PROGRAM IL
VAR
	RANGE_PG_PS1:RANGEJD;
	RANGE_PG_PS2:RANGEJD;
	RANGE_PG_PS3:RANGEJD;
	RANGE_PG_PS4:RANGEJD;
	RANGE_PG_PS5:RANGEJD;
	RANGE_PG_PS6:RANGEJD;
	RANGE_PG_PS7:RANGEJD;
	RANGE_PG_PS8:RANGEJD;
	RANGE_PG_PS9:RANGEJD;
	
	RANGE_MFC1:RANGEJD;
	RANGE_MFC2:RANGEJD;
	RANGE_MFC3:RANGEJD;
	RANGE_MFC4:RANGEJD;
	RANGE_MFC5:RANGEJD;
	RANGE_MFC6:RANGEJD;
	RANGE_MFC7:RANGEJD;
	RANGE_MFC8:RANGEJD;
	RANGE_MFC9:RANGEJD;
	
	RANGE_CHAMBER_HEATER1:RANGEJD;
	RANGE_CHAMBER_HEATER2:RANGEJD;
	RANGE_CHAMBER_HEATER3:RANGEJD;
	
	RANGE_LID_HEATER:RANGEJD;
	
	RANGE_STAGE1:RANGEJD;
	RANGE_STAGE2:RANGEJD;
	RANGE_STAGE3:RANGEJD;
	RANGE_STAGE4:RANGEJD;
	
	//INTERLOCK	
	TON_PrepareTransfer:TON;	
	TON_TransferWafer:TON;	
	TON_OpenGasValve:TON;	
	TON_CloseGasValve:TON;	
	TON_OpenCloseSlitValve:TON;
	
	ALWAYS_TRUE:BOOL:=TRUE;
END_VAR
VAR // added by the converter: edge detectors and wires of the graphical bodies
    _w1, _w2, _w3, _w4, _w5 : BOOL;
END_VAR

VALVE();
Temp();
SYS();
SPLC();
ACT_HEATER();
ACT_MFC();
ACT_PG_PS();

//TMP Pressure OUT OF RANGE
	IF GV.PMConfig.TurboN2Pressure	<=	GV.TurboN2PurgePressure
		THEN
		PM.INFO.Alarm.TurboN2PurgePressureOutOfRange:=TRUE;
		ELSE
		PM.INFO.Alarm.TurboN2PurgePressureOutOfRange:=FALSE;	
	END_IF
	
//PrepareTransfer TIMEOUT
	TON_PrepareTransfer(IN:= GV_IL.STATUS_PrepareTransfer, PT:=INT_TO_TIME(GV.PMConfig.PrepareTransferTimeout)*1000 , Q=> , ET=> );	
	IF TON_PrepareTransfer.Q
		THEN
		PM.INFO.Alarm.PrepareTransferTimerout:=TRUE;
		ELSE
		PM.INFO.Alarm.PrepareTransferTimerout:=FALSE;
	END_IF
	
//TransferWafer TIMEOUT
	TON_TransferWafer(IN:=GV_IL.STATUS_TransferWafer , PT:= INT_TO_TIME(GV.PMConfig.TransferWaferTimeout)*1000, Q=> , ET=> );
	IF TON_TransferWafer.Q
		THEN
		PM.INFO.Alarm.TransferWaferTimeout:=TRUE;
		ELSE
		PM.INFO.Alarm.TransferWaferTimeout:=FALSE;	
	END_IF
	
//OpenGasValve TIMEOUT
	TON_OpenGasValve(IN:=GV_IL.STATUS_OpenGasValve , PT:= INT_TO_TIME(GV.PMConfig.OpenGasValveTimeout)*1000, Q=> , ET=> );
	IF TON_OpenGasValve.Q
		THEN
		PM.INFO.Alarm.OpenGasValveTimeout:=TRUE;
		ELSE 
		PM.INFO.Alarm.OpenGasValveTimeout:=FALSE;
	END_IF
	
//CloseGasValve TIMEOUT
	TON_CloseGasValve(IN:=GV_IL.STATUS_CloseGasValve , PT:= INT_TO_TIME(GV.PMConfig.CloseGasValveTimeout)*1000, Q=> , ET=> );
	IF TON_CloseGasValve.Q
		THEN
		PM.INFO.Alarm.CloseGasValveTimeout:=TRUE;
		ELSE
		PM.INFO.Alarm.CloseGasValveTimeout:=FALSE;
	END_IF
	
//OpenCloseSlitValve TIMEOUT
	TON_OpenCloseSlitValve(IN:=GV_IL.STATUS_OpenCloseSlitValve , PT:= INT_TO_TIME(GV.PMConfig.OpenCloseSlitValveTimeout)*1000, Q=> , ET=> );
	IF TON_OpenCloseSlitValve.Q
		THEN
		PM.INFO.Alarm.OpenCloseSlitValveTimeout:=TRUE;
		ELSE
		PM.INFO.Alarm.OpenCloseSlitValveTimeout:=FALSE;	
	END_IF
	
	
//PRESSURE ALARM
	//PM.INFO.Alarm.PRESSURE:=
	
//ALARM OR WARNING OCCUR
	GV.ALARM_OCC:=NOT (
				 	//PM.INFO.Alarm.PRESSURE
					PM.INFO.Alarm.MFC1	
				AND PM.INFO.Alarm.MFC2	
				AND	PM.INFO.Alarm.MFC3
				AND PM.INFO.Alarm.MFC4	
				AND PM.INFO.Alarm.MFC5	
				AND PM.INFO.Alarm.MFC6
				AND PM.INFO.Alarm.MFC7	
				AND PM.INFO.Alarm.MFC8	
				AND PM.INFO.Alarm.MFC9
				AND PM.INFO.Alarm.WALL_TEMP	
				AND PM.INFO.Alarm.LID_TEMP	
				AND PM.INFO.Alarm.STAGE_TEMP1
				AND PM.INFO.Alarm.STAGE_TEMP2
				AND PM.INFO.Alarm.STAGE_TEMP3
				AND PM.INFO.Alarm.STAGE_TEMP4
				//AND PM.INFO.Alarm.Gas1FlowPressureOutOfRange
				//AND PM.INFO.Alarm.Gas2FlowPressureOutOfRange
				//AND PM.INFO.Alarm.Gas3FlowPressureOutOfRange
				//AND PM.INFO.Alarm.Gas4FlowPressureOutOfRange
				//AND PM.INFO.Alarm.Gas5FlowPressureOutOfRange
				//AND PM.INFO.Alarm.Gas6FlowPressureOutOfRange
				//AND PM.INFO.Alarm.TurboN2PurgePressureOutOfRange
				//AND PM.INFO.Alarm.PrepareTransferTimerout
				//AND PM.INFO.Alarm.TransferWaferTimeout
				//AND PM.INFO.Alarm.OpenGasValveTimeout
				//AND PM.INFO.Alarm.CloseGasValveTimeout
				//AND PM.INFO.Alarm.OpenCloseSlitValveTimeout
				//AND PM.INFO.Alarm.ATMCheckTimeout
				//AND PM.INFO.Alarm.DRY_PUMP
				//AND PM.INFO.Alarm.PENDULUM_VALVE
				//AND PM.INFO.Alarm.TURBO_PUMP
				AND (PM.INFO.Alarm.TOLERANCE_PRESSURE				
				AND PM.INFO.Alarm.TOLERANCE_MFC1
				AND PM.INFO.Alarm.TOLERANCE_MFC2
				AND PM.INFO.Alarm.TOLERANCE_MFC3
				AND PM.INFO.Alarm.TOLERANCE_MFC4
				AND PM.INFO.Alarm.TOLERANCE_MFC5
				AND PM.INFO.Alarm.TOLERANCE_MFC6
				AND PM.INFO.Alarm.TOLERANCE_MFC7
				AND PM.INFO.Alarm.TOLERANCE_MFC8
				AND PM.INFO.Alarm.TOLERANCE_MFC9
				AND PM.INFO.Alarm.TOLERANCE_WALL_TEMP
				AND PM.INFO.Alarm.TOLERANCE_LID_TEMP
				AND PM.INFO.Alarm.TOLERANCE_STAGE_TEMP1
				AND PM.INFO.Alarm.TOLERANCE_STAGE_TEMP2
				AND PM.INFO.Alarm.TOLERANCE_STAGE_TEMP3
				AND PM.INFO.Alarm.TOLERANCE_STAGE_TEMP4)
				);

	GV.WARNING_OCC:=NOT (
					//PM.INFO.Warning.PRESSURE					
					PM.INFO.Warning.MFC1
				AND PM.INFO.Warning.MFC2
				AND PM.INFO.Warning.MFC3
				AND PM.INFO.Warning.MFC4
				AND PM.INFO.Warning.MFC5
				AND PM.INFO.Warning.MFC6
				AND PM.INFO.Warning.MFC7
				AND PM.INFO.Warning.MFC8
				AND PM.INFO.Warning.MFC9
				AND PM.INFO.Warning.WALL_TEMP
				AND PM.INFO.Warning.LID_TEMP
				AND PM.INFO.Warning.STAGE_TEMP1
				AND PM.INFO.Warning.STAGE_TEMP2
				AND PM.INFO.Warning.STAGE_TEMP3
				AND PM.INFO.Warning.STAGE_TEMP4
				//AND PM.INFO.Warning.Gas1FlowPressureOutOfRange
				//AND PM.INFO.Warning.Gas2FlowPressureOutOfRange
				//AND PM.INFO.Warning.Gas3FlowPressureOutOfRange
				//AND PM.INFO.Warning.Gas4FlowPressureOutOfRange
				//AND PM.INFO.Warning.Gas5FlowPressureOutOfRange
				//AND PM.INFO.Warning.Gas6FlowPressureOutOfRange
				//AND PM.INFO.Warning.OpenCloseSlitValveTimeout
				AND (PM.INFO.Warning.TOLERANCE_PRESSURE
				AND PM.INFO.Warning.TOLERANCE_MFC1
				AND PM.INFO.Warning.TOLERANCE_MFC2
				AND PM.INFO.Warning.TOLERANCE_MFC3
				AND PM.INFO.Warning.TOLERANCE_MFC4
				AND PM.INFO.Warning.TOLERANCE_MFC5
				AND PM.INFO.Warning.TOLERANCE_MFC6
				AND PM.INFO.Warning.TOLERANCE_MFC7
				AND PM.INFO.Warning.TOLERANCE_MFC8
				AND PM.INFO.Warning.TOLERANCE_MFC9
				AND PM.INFO.Warning.TOLERANCE_WALL_TEMP
				AND PM.INFO.Warning.TOLERANCE_LID_TEMP
				AND PM.INFO.Warning.TOLERANCE_STAGE_TEMP1
				AND PM.INFO.Warning.TOLERANCE_STAGE_TEMP2
				AND PM.INFO.Warning.TOLERANCE_STAGE_TEMP3
				AND PM.INFO.Warning.TOLERANCE_STAGE_TEMP4)
				);

ACTION ACT_HEATER:
//CHAMBER HEATER
	RANGE_CHAMBER_HEATER1(
	ENABLE:= GV.ChamberHeater.HeaterTolerance_Enable,
	SV:= REAL_TO_LREAL(GV.AO.Chamber_Temp1_SV),
	PV:= REAL_TO_LREAL( GV.AI.Chamber_Temp1), 
	RANGE_ALARM_H:= ANY_TO_REAL(GV.ChamberHeater.HeaterAlarmRange.SV), 
	RANGE_ALARM_L:= ANY_TO_LREAL(GV.ChamberHeater.HeaterAlarmRange.SV), 
	RANGE_WARNING_H:= ANY_TO_LREAL(GV.ChamberHeater.HeaterWarningRange.SV), 
	RANGE_WARNING_L:= ANY_TO_LREAL(GV.ChamberHeater.HeaterWarningRange.SV), 
	TIME_ALARM:= ANY_TO_LREAL(GV.ChamberHeater.HeaterAlarmTime.SV), 
	TIME_WARNING:= ANY_TO_LREAL(GV.ChamberHeater.HeaterWarningTime.SV), 
	ALARM=> , 
	WARNING=> );
	
	RANGE_CHAMBER_HEATER2(
	ENABLE:= GV.ChamberHeater.HeaterTolerance_Enable,
	SV:= REAL_TO_LREAL(GV.AO.Chamber_Temp2_SV),
	PV:= REAL_TO_LREAL( GV.AI.Chamber_Temp2), 
	RANGE_ALARM_H:= ANY_TO_LREAL(GV.ChamberHeater.HeaterAlarmRange.SV), 
	RANGE_ALARM_L:= ANY_TO_LREAL(GV.ChamberHeater.HeaterAlarmRange.SV), 
	RANGE_WARNING_H:= ANY_TO_LREAL(GV.ChamberHeater.HeaterWarningRange.SV), 
	RANGE_WARNING_L:= ANY_TO_LREAL(GV.ChamberHeater.HeaterWarningRange.SV), 
	TIME_ALARM:= ANY_TO_LREAL(GV.ChamberHeater.HeaterAlarmTime.SV), 
	TIME_WARNING:= ANY_TO_LREAL(GV.ChamberHeater.HeaterWarningTime.SV), 
	ALARM=> , 
	WARNING=> );
	
	RANGE_CHAMBER_HEATER3(
	ENABLE:= GV.ChamberHeater.HeaterTolerance_Enable,
	SV:= REAL_TO_LREAL(GV.AO.Chamber_Temp3_SV),
	PV:= REAL_TO_LREAL( GV.AI.Chamber_Temp3), 
	RANGE_ALARM_H:= ANY_TO_LREAL(GV.ChamberHeater.HeaterAlarmRange.SV), 
	RANGE_ALARM_L:= ANY_TO_LREAL(GV.ChamberHeater.HeaterAlarmRange.SV), 
	RANGE_WARNING_H:= ANY_TO_LREAL(GV.ChamberHeater.HeaterWarningRange.SV), 
	RANGE_WARNING_L:= ANY_TO_LREAL(GV.ChamberHeater.HeaterWarningRange.SV), 
	TIME_ALARM:= ANY_TO_LREAL(GV.ChamberHeater.HeaterAlarmTime.SV), 
	TIME_WARNING:= ANY_TO_LREAL(GV.ChamberHeater.HeaterWarningTime.SV), 
	ALARM=> , 
	WARNING=> );
	
	PM.INFO.Alarm.WALL_TEMP:=	RANGE_CHAMBER_HEATER1.ALARM 
							AND RANGE_CHAMBER_HEATER2.ALARM 
							AND RANGE_CHAMBER_HEATER3.ALARM
								;
	PM.INFO.Warning.WALL_TEMP:=	RANGE_CHAMBER_HEATER1.WARNING 
							AND RANGE_CHAMBER_HEATER2.WARNING 
							AND RANGE_CHAMBER_HEATER3.WARNING
								;
//LID HEATER
	RANGE_LID_HEATER(
	ENABLE:= GV.LidHeater.HeaterTolerance_Enable,
	SV:= REAL_TO_LREAL(GV.AO.LID_Temp_SV),
	PV:= REAL_TO_LREAL( GV.AI.Lid_Temp), 
	RANGE_ALARM_H:= ANY_TO_LREAL(GV.LidHeater.HeaterAlarmRange.SV), 
	RANGE_ALARM_L:= ANY_TO_LREAL(GV.LidHeater.HeaterAlarmRange.SV), 
	RANGE_WARNING_H:= ANY_TO_LREAL(GV.LidHeater.HeaterWarningRange.SV), 
	RANGE_WARNING_L:= ANY_TO_LREAL(GV.LidHeater.HeaterWarningRange.SV), 
	TIME_ALARM:= ANY_TO_LREAL(GV.LidHeater.HeaterAlarmTime.SV), 
	TIME_WARNING:= ANY_TO_LREAL(GV.LidHeater.HeaterWarningTime.SV), 
	ALARM=> , 
	WARNING=> );
	
	PM.INFO.Alarm.LID_TEMP	:=	RANGE_LID_HEATER.ALARM ;
	PM.INFO.Warning.LID_TEMP:=	RANGE_LID_HEATER.WARNING;
	
//STAGE HEATER
	RANGE_STAGE1(
	ENABLE:= GV.STAGE.HeaterTolerance_Enable,
	SV:= REAL_TO_LREAL(GV.AO.Stage_Temp1_SV),
	PV:= REAL_TO_LREAL( GV.AI.Stage_Temp1), 
	RANGE_ALARM_H:= ANY_TO_LREAL(GV.STAGE.HeaterAlarmRange.SV), 
	RANGE_ALARM_L:= ANY_TO_LREAL(GV.STAGE.HeaterAlarmRange.SV), 
	RANGE_WARNING_H:= ANY_TO_LREAL(GV.STAGE.HeaterWarningRange.SV), 
	RANGE_WARNING_L:= ANY_TO_LREAL(GV.STAGE.HeaterWarningRange.SV), 
	TIME_ALARM:= ANY_TO_LREAL(GV.STAGE.HeaterAlarmTime.SV), 
	TIME_WARNING:= ANY_TO_LREAL(GV.STAGE.HeaterWarningTime.SV), 
	ALARM=> , 
	WARNING=> );
	
	PM.INFO.Alarm.STAGE_TEMP1:=RANGE_STAGE1.ALARM;
	PM.INFO.Warning.STAGE_TEMP1:=RANGE_STAGE1.WARNING;

	RANGE_STAGE2(
	ENABLE:= GV.STAGE.HeaterTolerance_Enable,
	SV:= REAL_TO_LREAL(GV.AO.Stage_Temp2_SV),
	PV:= REAL_TO_LREAL( GV.AI.Stage_Temp2), 
	RANGE_ALARM_H:= ANY_TO_LREAL(GV.STAGE.HeaterAlarmRange.SV), 
	RANGE_ALARM_L:= ANY_TO_LREAL(GV.STAGE.HeaterAlarmRange.SV), 
	RANGE_WARNING_H:= ANY_TO_LREAL(GV.STAGE.HeaterWarningRange.SV), 
	RANGE_WARNING_L:= ANY_TO_LREAL(GV.STAGE.HeaterWarningRange.SV), 
	TIME_ALARM:= ANY_TO_LREAL(GV.STAGE.HeaterAlarmTime.SV), 
	TIME_WARNING:= ANY_TO_LREAL(GV.STAGE.HeaterWarningTime.SV), 
	ALARM=> , 
	WARNING=> );
	
	PM.INFO.Alarm.STAGE_TEMP2:=RANGE_STAGE2.ALARM;
	PM.INFO.Warning.STAGE_TEMP2:=RANGE_STAGE2.WARNING;
	
	RANGE_STAGE3(
	ENABLE:= GV.STAGE.HeaterTolerance_Enable,
	SV:= REAL_TO_LREAL(GV.AO.Stage_Temp3_SV),
	PV:= REAL_TO_LREAL( GV.AI.Stage_Temp3), 
	RANGE_ALARM_H:= ANY_TO_LREAL(GV.STAGE.HeaterAlarmRange.SV), 
	RANGE_ALARM_L:= ANY_TO_LREAL(GV.STAGE.HeaterAlarmRange.SV), 
	RANGE_WARNING_H:= ANY_TO_LREAL(GV.STAGE.HeaterWarningRange.SV), 
	RANGE_WARNING_L:= ANY_TO_LREAL(GV.STAGE.HeaterWarningRange.SV), 
	TIME_ALARM:= ANY_TO_LREAL(GV.STAGE.HeaterAlarmTime.SV), 
	TIME_WARNING:= ANY_TO_LREAL(GV.STAGE.HeaterWarningTime.SV), 
	ALARM=> , 
	WARNING=> );
	
	PM.INFO.Alarm.STAGE_TEMP3:=RANGE_STAGE3.ALARM;
	PM.INFO.Warning.STAGE_TEMP3:=RANGE_STAGE3.WARNING;
	
	RANGE_STAGE4(
	ENABLE:= GV.STAGE.HeaterTolerance_Enable,
	SV:= REAL_TO_LREAL(GV.AO.Stage_Temp4_SV),
	PV:= REAL_TO_LREAL( GV.AI.Stage_Temp4), 
	RANGE_ALARM_H:= ANY_TO_LREAL(GV.STAGE.HeaterAlarmRange.SV), 
	RANGE_ALARM_L:= ANY_TO_LREAL(GV.STAGE.HeaterAlarmRange.SV), 
	RANGE_WARNING_H:= ANY_TO_LREAL(GV.STAGE.HeaterWarningRange.SV), 
	RANGE_WARNING_L:= ANY_TO_LREAL(GV.STAGE.HeaterWarningRange.SV), 
	TIME_ALARM:= ANY_TO_LREAL(GV.STAGE.HeaterAlarmTime.SV), 
	TIME_WARNING:= ANY_TO_LREAL(GV.STAGE.HeaterWarningTime.SV), 
	ALARM=> , 
	WARNING=> );
	
	PM.INFO.Alarm.STAGE_TEMP4:=RANGE_STAGE4.ALARM;
	PM.INFO.Warning.STAGE_TEMP4:=RANGE_STAGE4.WARNING;
END_ACTION

ACTION ACT_MFC:
RANGE_MFC1(
	ENABLE:= GV.Mfcgas1.EnableAlarm AND GV.Mfcgas1.Enable,
	SV:= REAL_TO_LREAL(GV.AO.MFC1_Flow_Setpoint),
	PV:= REAL_TO_LREAL( GV.AI.MFC1_Flow), 
	RANGE_ALARM_H:= GV.Mfcgas1.AlarmRange.SV, 
	RANGE_ALARM_L:= GV.Mfcgas1.AlarmRange.SV, 
	RANGE_WARNING_H:= GV.Mfcgas1.WarningRange.SV, 
	RANGE_WARNING_L:= GV.Mfcgas1.WarningRange.SV, 
	TIME_ALARM:= GV.Mfcgas1.AlarmTime.SV, 
	TIME_WARNING:= GV.Mfcgas1.WarningTime.SV, 
	ALARM=> , 
	WARNING=> );
	
	RANGE_MFC2(
	ENABLE:= GV.Mfcgas2.EnableAlarm AND GV.Mfcgas2.Enable, 
	SV:= REAL_TO_LREAL(GV.AO.MFC2_Flow_Setpoint),
	PV:= REAL_TO_LREAL( GV.AI.MFC2_Flow), 
	RANGE_ALARM_H:= GV.Mfcgas2.AlarmRange.SV, 
	RANGE_ALARM_L:= GV.Mfcgas2.AlarmRange.SV, 
	RANGE_WARNING_H:= GV.Mfcgas2.WarningRange.SV, 
	RANGE_WARNING_L:= GV.Mfcgas2.WarningRange.SV, 
	TIME_ALARM:= GV.Mfcgas2.AlarmTime.SV, 
	TIME_WARNING:= GV.Mfcgas2.WarningTime.SV, 
	ALARM=> , 
	WARNING=> );

	RANGE_MFC3(	
	ENABLE:= GV.Mfcgas3.EnableAlarm AND GV.Mfcgas3.Enable, 
	SV:= REAL_TO_LREAL(GV.AO.MFC3_Flow_Setpoint),
	PV:= REAL_TO_LREAL( GV.AI.MFC3_Flow), 
	RANGE_ALARM_H:= GV.Mfcgas3.AlarmRange.SV, 
	RANGE_ALARM_L:= GV.Mfcgas3.AlarmRange.SV, 
	RANGE_WARNING_H:= GV.Mfcgas3.WarningRange.SV, 
	RANGE_WARNING_L:= GV.Mfcgas3.WarningRange.SV, 
	TIME_ALARM:= GV.Mfcgas3.AlarmTime.SV, 
	TIME_WARNING:= GV.Mfcgas3.WarningTime.SV,  
	ALARM=> , 
	WARNING=> );

	RANGE_MFC4(	
	ENABLE:= GV.Mfcgas4.EnableAlarm AND GV.Mfcgas4.Enable, 
	SV:= REAL_TO_LREAL(GV.AO.MFC4_Flow_Setpoint),
	PV:= REAL_TO_LREAL( GV.AI.MFC4_Flow), 
	RANGE_ALARM_H:= GV.Mfcgas4.AlarmRange.SV, 
	RANGE_ALARM_L:= GV.Mfcgas4.AlarmRange.SV, 
	RANGE_WARNING_H:= GV.Mfcgas4.WarningRange.SV, 
	RANGE_WARNING_L:= GV.Mfcgas4.WarningRange.SV, 
	TIME_ALARM:= GV.Mfcgas4.AlarmTime.SV, 
	TIME_WARNING:= GV.Mfcgas4.WarningTime.SV, 
	ALARM=> , 
	WARNING=> );
	
	RANGE_MFC5(	
	ENABLE:= GV.Mfcgas5.EnableAlarm AND GV.Mfcgas5.Enable, 
	SV:= REAL_TO_LREAL(GV.AO.MFC5_Flow_Setpoint),
	PV:= REAL_TO_LREAL( GV.AI.MFC5_Flow), 
	RANGE_ALARM_H:= GV.Mfcgas5.AlarmRange.SV, 
	RANGE_ALARM_L:= GV.Mfcgas5.AlarmRange.SV, 
	RANGE_WARNING_H:= GV.Mfcgas5.WarningRange.SV, 
	RANGE_WARNING_L:= GV.Mfcgas5.WarningRange.SV, 
	TIME_ALARM:= GV.Mfcgas5.AlarmTime.SV, 
	TIME_WARNING:= GV.Mfcgas5.WarningTime.SV, 
	ALARM=> , 
	WARNING=> );

	RANGE_MFC6(	
	ENABLE:= GV.Mfcgas6.EnableAlarm AND GV.Mfcgas6.Enable, 
	SV:= REAL_TO_LREAL(GV.AO.MFC6_Flow_Setpoint),
	PV:= REAL_TO_LREAL( GV.AI.MFC6_Flow), 
	RANGE_ALARM_H:= GV.Mfcgas6.AlarmRange.SV, 
	RANGE_ALARM_L:= GV.Mfcgas6.AlarmRange.SV, 
	RANGE_WARNING_H:= GV.Mfcgas6.WarningRange.SV, 
	RANGE_WARNING_L:= GV.Mfcgas6.WarningRange.SV, 
	TIME_ALARM:= GV.Mfcgas6.AlarmTime.SV, 
	TIME_WARNING:= GV.Mfcgas6.WarningTime.SV,  
	ALARM=> , 
	WARNING=> );

	RANGE_MFC7(	
	ENABLE:= GV.Mfcgas7.EnableAlarm AND GV.Mfcgas7.Enable, 
	SV:= REAL_TO_LREAL(GV.AO.MFC7_Flow_Setpoint),
	PV:= REAL_TO_LREAL( GV.AI.MFC7_Flow), 
	RANGE_ALARM_H:= GV.Mfcgas7.AlarmRange.SV, 
	RANGE_ALARM_L:= GV.Mfcgas7.AlarmRange.SV, 
	RANGE_WARNING_H:= GV.Mfcgas7.WarningRange.SV, 
	RANGE_WARNING_L:= GV.Mfcgas7.WarningRange.SV, 
	TIME_ALARM:= GV.Mfcgas7.AlarmTime.SV, 
	TIME_WARNING:= GV.Mfcgas7.WarningTime.SV, 
	ALARM=> , 
	WARNING=> );
(*
	RANGE_MFC8(	
	ENABLE:= GV.Mfcgas8.EnableAlarm AND GV.Mfcgas8.Enable, 
	PV:= REAL_TO_LREAL( GV.AI.MFC8_Flow), 
	RANGE_ALARM_H:= GV.Mfcgas8.AlarmRange.MaxSV, 
	RANGE_ALARM_L:= 0, 
	RANGE_WARNING_H:= GV.Mfcgas8.WarningRange.MaxSV, 
	RANGE_WARNING_L:= 0, 
	TIME_ALARM:= GV.Mfcgas8.AlarmTime.SV, 
	TIME_WARNING:= GV.Mfcgas8.WarningTime.SV, 
	ALARM=> , 
	WARNING=> );

	RANGE_MFC9(	
	ENABLE:= GV.Mfcgas9.EnableAlarm AND GV.Mfcgas9.Enable, 
	PV:= REAL_TO_LREAL( GV.AI.MFC9_Flow), 
	RANGE_ALARM_H:= GV.Mfcgas9.AlarmRange.MaxSV, 
	RANGE_ALARM_L:= 0, 
	RANGE_WARNING_H:= GV.Mfcgas9.WarningRange.MaxSV, 
	RANGE_WARNING_L:= 0, 
	TIME_ALARM:= GV.Mfcgas9.AlarmTime.SV, 
	TIME_WARNING:= GV.Mfcgas9.WarningTime.SV, 
	ALARM=> , 
	WARNING=> );
*)	
	
	PM.Info.Alarm.MFC1:=  RANGE_MFC1.ALARM;
	PM.INFO.Alarm.MFC2:=  RANGE_MFC2.ALARM;
	PM.INFO.Alarm.MFC3:=  RANGE_MFC3.ALARM;
	PM.INFO.Alarm.MFC4:=  RANGE_MFC4.ALARM;
	PM.INFO.Alarm.MFC5:=  RANGE_MFC5.ALARM;
	PM.INFO.Alarm.MFC6:=  RANGE_MFC6.ALARM;
	PM.INFO.Alarm.MFC7:=  RANGE_MFC7.ALARM;
	PM.INFO.Alarm.MFC8:=  RANGE_MFC8.ALARM OR TRUE;
	PM.INFO.Alarm.MFC9:=  RANGE_MFC9.ALARM OR TRUE;
	
	PM.INFO.warning.MFC1:=  RANGE_MFC1.warning;
	PM.INFO.warning.MFC2:=  RANGE_MFC2.warning;
	PM.INFO.warning.MFC3:=  RANGE_MFC3.warning;
	PM.INFO.warning.MFC4:=  RANGE_MFC4.warning;
	PM.INFO.warning.MFC5:=  RANGE_MFC5.warning;
	PM.INFO.warning.MFC6:=  RANGE_MFC6.warning;
	PM.INFO.warning.MFC7:=  RANGE_MFC7.warning;
	PM.INFO.warning.MFC8:=  RANGE_MFC8.warning OR TRUE;
	PM.INFO.warning.MFC9:=  RANGE_MFC9.warning OR TRUE;
END_ACTION

ACTION ACT_PG_PS:
RANGE_PG_PS1(
	ENABLE:=TRUE,
	SV:= 270,
	PV:= GV.AI.PG_PS1_VALUE, 
	RANGE_ALARM_H:= GV.PMConfig.GasFlowPressureAlarmRange, 
	RANGE_ALARM_L:= GV.PMConfig.GasFlowPressureAlarmRange, 
	RANGE_WARNING_H:= GV.PMConfig.GasFlowPressureWarningRange, 
	RANGE_WARNING_L:= GV.PMConfig.GasFlowPressureWarningRange, 
	TIME_ALARM:= GV.PMConfig.GasFlowPressureAlarmTime, 
	TIME_WARNING:= GV.PMConfig.GasFlowPressureWarningTime, 
	ALARM=> , 
	WARNING=> );
	
	RANGE_PG_PS2(
	ENABLE:=TRUE,
	SV:= 270 ,
	PV:= GV.AI.PG_PS2_VALUE, 
	RANGE_ALARM_H:= GV.PMConfig.GasFlowPressureAlarmRange, 
	RANGE_ALARM_L:= GV.PMConfig.GasFlowPressureAlarmRange, 
	RANGE_WARNING_H:= GV.PMConfig.GasFlowPressureWarningRange, 
	RANGE_WARNING_L:= GV.PMConfig.GasFlowPressureWarningRange, 
	TIME_ALARM:= GV.PMConfig.GasFlowPressureAlarmTime, 
	TIME_WARNING:= GV.PMConfig.GasFlowPressureWarningTime, 
	ALARM=> , 
	WARNING=> );
	
	RANGE_PG_PS3(
	ENABLE:=TRUE,
	SV:= 270 ,
	PV:= GV.AI.PG_PS3_VALUE, 
	RANGE_ALARM_H:= GV.PMConfig.GasFlowPressureAlarmRange, 
	RANGE_ALARM_L:= GV.PMConfig.GasFlowPressureAlarmRange, 
	RANGE_WARNING_H:= GV.PMConfig.GasFlowPressureWarningRange, 
	RANGE_WARNING_L:= GV.PMConfig.GasFlowPressureWarningRange, 
	TIME_ALARM:= GV.PMConfig.GasFlowPressureAlarmTime, 
	TIME_WARNING:= GV.PMConfig.GasFlowPressureWarningTime, 
	ALARM=> , 
	WARNING=> );
	
	RANGE_PG_PS4(
	ENABLE:=TRUE,
	SV:=25,
	PV:= GV.AI.PG_PS4_VALUE, 
	RANGE_ALARM_H:= GV.PMConfig.GasFlowPressureAlarmRange, 
	RANGE_ALARM_L:= GV.PMConfig.GasFlowPressureAlarmRange, 
	RANGE_WARNING_H:= GV.PMConfig.GasFlowPressureWarningRange, 
	RANGE_WARNING_L:= GV.PMConfig.GasFlowPressureWarningRange, 
	TIME_ALARM:= GV.PMConfig.GasFlowPressureAlarmTime, 
	TIME_WARNING:= GV.PMConfig.GasFlowPressureWarningTime, 
	ALARM=> , 
	WARNING=> );
	
	RANGE_PG_PS5(
	ENABLE:=TRUE,
	SV:= 270,
	PV:= GV.AI.PG_PS5_VALUE, 
	RANGE_ALARM_H:= GV.PMConfig.GasFlowPressureAlarmRange, 
	RANGE_ALARM_L:= GV.PMConfig.GasFlowPressureAlarmRange, 
	RANGE_WARNING_H:= GV.PMConfig.GasFlowPressureWarningRange, 
	RANGE_WARNING_L:= GV.PMConfig.GasFlowPressureWarningRange, 
	TIME_ALARM:= GV.PMConfig.GasFlowPressureAlarmTime, 
	TIME_WARNING:= GV.PMConfig.GasFlowPressureWarningTime, 
	ALARM=> , 
	WARNING=> );
	
	RANGE_PG_PS6(
	ENABLE:=TRUE,
	SV:=270,
	PV:= GV.AI.PG_PS6_VALUE, 
	RANGE_ALARM_H:= GV.PMConfig.GasFlowPressureAlarmRange, 
	RANGE_ALARM_L:= GV.PMConfig.GasFlowPressureAlarmRange, 
	RANGE_WARNING_H:= GV.PMConfig.GasFlowPressureWarningRange, 
	RANGE_WARNING_L:= GV.PMConfig.GasFlowPressureWarningRange, 
	TIME_ALARM:= GV.PMConfig.GasFlowPressureAlarmTime, 
	TIME_WARNING:= GV.PMConfig.GasFlowPressureWarningTime, 
	ALARM=> , 
	WARNING=> );
	
	RANGE_PG_PS7(
	ENABLE:=TRUE,
	PV:= GV.AI.PG_PS7_VALUE, 
	RANGE_ALARM_H:= GV.PMConfig.GasFlowPressureAlarmRange, 
	RANGE_ALARM_L:= GV.PMConfig.GasFlowPressureAlarmRange, 
	RANGE_WARNING_H:= GV.PMConfig.GasFlowPressureWarningRange, 
	RANGE_WARNING_L:= GV.PMConfig.GasFlowPressureWarningRange, 
	TIME_ALARM:= GV.PMConfig.GasFlowPressureAlarmTime, 
	TIME_WARNING:= GV.PMConfig.GasFlowPressureWarningTime, 
	ALARM=> , 
	WARNING=> );
	
	RANGE_PG_PS8(
	ENABLE:=TRUE,
	PV:= GV.AI.PG_PS8_VALUE, 
	RANGE_ALARM_H:= GV.PMConfig.GasFlowPressureAlarmRange, 
	RANGE_ALARM_L:= GV.PMConfig.GasFlowPressureAlarmRange, 
	RANGE_WARNING_H:= GV.PMConfig.GasFlowPressureWarningRange, 
	RANGE_WARNING_L:= GV.PMConfig.GasFlowPressureWarningRange, 
	TIME_ALARM:= GV.PMConfig.GasFlowPressureAlarmTime, 
	TIME_WARNING:= GV.PMConfig.GasFlowPressureWarningTime, 
	ALARM=> , 
	WARNING=> );
	
	RANGE_PG_PS9(
	ENABLE:=TRUE,
	PV:= GV.AI.PG_PS9_VALUE, 
	RANGE_ALARM_H:= GV.PMConfig.GasFlowPressureAlarmRange, 
	RANGE_ALARM_L:= GV.PMConfig.GasFlowPressureAlarmRange, 
	RANGE_WARNING_H:= GV.PMConfig.GasFlowPressureWarningRange, 
	RANGE_WARNING_L:= GV.PMConfig.GasFlowPressureWarningRange, 
	TIME_ALARM:= GV.PMConfig.GasFlowPressureAlarmTime, 
	TIME_WARNING:= GV.PMConfig.GasFlowPressureWarningTime, 
	ALARM=> , 
	WARNING=> );
	
	PM.INFO.Alarm.Gas1FlowPressureOutOfRange:=  RANGE_PG_PS1.ALARM;
	PM.INFO.Alarm.Gas2FlowPressureOutOfRange:=  RANGE_PG_PS2.ALARM;
	PM.INFO.Alarm.Gas3FlowPressureOutOfRange:=  RANGE_PG_PS3.ALARM;	
	PM.INFO.Alarm.Gas4FlowPressureOutOfRange:=  RANGE_PG_PS4.ALARM OR TRUE;
	PM.INFO.Alarm.Gas5FlowPressureOutOfRange:=  RANGE_PG_PS5.ALARM;
	PM.INFO.Alarm.Gas6FlowPressureOutOfRange:=  RANGE_PG_PS6.ALARM;
	//PM.INFO.Alarm.Gas7FlowPressureOutOfRange:=  RANGE_PG_PS7.ALARM;
	//PM.INFO.Alarm.Gas8FlowPressureOutOfRange:=  RANGE_PG_PS8.ALARM;
	//PM.INFO.Alarm.Gas9FlowPressureOutOfRange:=  RANGE_PG_PS9.ALARM;

	PM.INFO.warning.Gas1FlowPressureOutOfRange:=  RANGE_PG_PS1.warning;
	PM.INFO.warning.Gas2FlowPressureOutOfRange:=  RANGE_PG_PS2.warning;
	PM.INFO.warning.Gas3FlowPressureOutOfRange:=  RANGE_PG_PS3.warning;
	PM.INFO.warning.Gas4FlowPressureOutOfRange:=  RANGE_PG_PS4.warning;
	PM.INFO.warning.Gas5FlowPressureOutOfRange:=  RANGE_PG_PS5.warning;
	PM.INFO.warning.Gas6FlowPressureOutOfRange:=  RANGE_PG_PS6.warning;
	//PM.INFO.warning.Gas7FlowPressureOutOfRange:=  RANGE_PG_PS7.warning;
	//PM.INFO.warning.Gas8FlowPressureOutOfRange:=  RANGE_PG_PS8.warning;
	//PM.INFO.warning.Gas9FlowPressureOutOfRange:=  RANGE_PG_PS9.warning;
END_ACTION

ACTION SPLC:
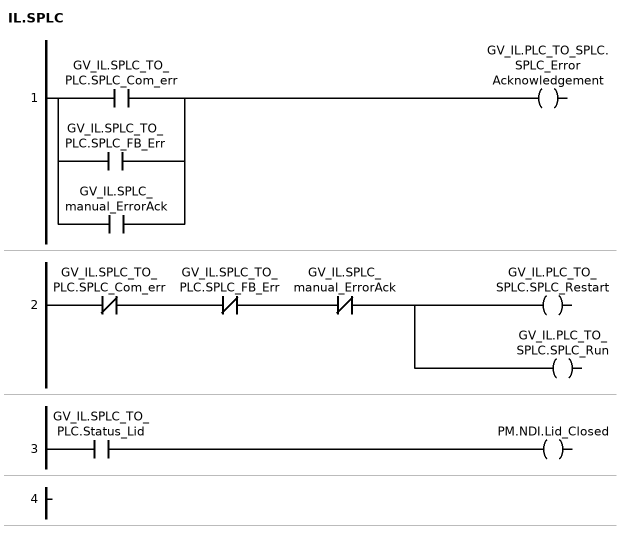
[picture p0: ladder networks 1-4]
// NETWORK 1
GV_IL.PLC_TO_SPLC.SPLC_ErrorAcknowledgement := GV_IL.SPLC_TO_PLC.SPLC_Com_err OR GV_IL.SPLC_TO_PLC.SPLC_FB_Err OR GV_IL.SPLC_manual_ErrorAck;

// NETWORK 2
_w1 := NOT GV_IL.SPLC_TO_PLC.SPLC_Com_err AND NOT GV_IL.SPLC_TO_PLC.SPLC_FB_Err AND NOT GV_IL.SPLC_manual_ErrorAck;
GV_IL.PLC_TO_SPLC.SPLC_Restart := _w1;
GV_IL.PLC_TO_SPLC.SPLC_Run := _w1;

// NETWORK 3
PM.NDI.Lid_Closed := GV_IL.SPLC_TO_PLC.Status_Lid;

// NETWORK 4
END_ACTION

ACTION SYS:
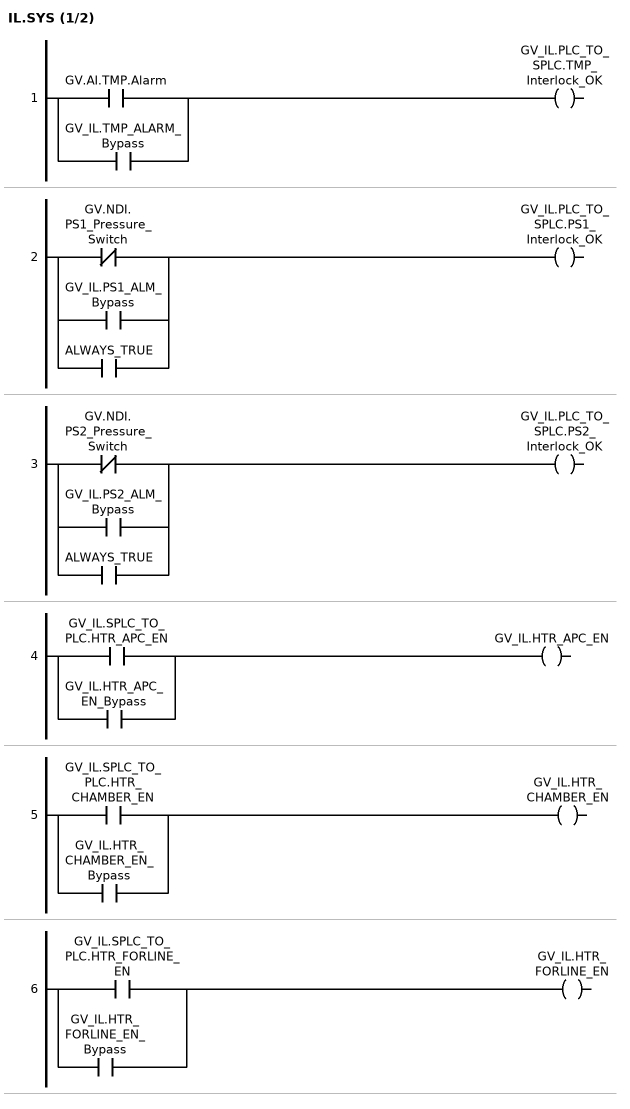
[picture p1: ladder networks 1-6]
// NETWORK 1
GV_IL.PLC_TO_SPLC.TMP_Interlock_OK := GV.AI.TMP.Alarm OR GV_IL.TMP_ALARM_Bypass;

// NETWORK 2
GV_IL.PLC_TO_SPLC.PS1_Interlock_OK := NOT (GV.NDI.	PS1_Pressure_Switch) OR GV_IL.PS1_ALM_Bypass OR ALWAYS_TRUE;

// NETWORK 3
GV_IL.PLC_TO_SPLC.PS2_Interlock_OK := NOT (GV.NDI.	PS2_Pressure_Switch) OR GV_IL.PS2_ALM_Bypass OR ALWAYS_TRUE;

// NETWORK 4
GV_IL.HTR_APC_EN := GV_IL.SPLC_TO_PLC.HTR_APC_EN OR GV_IL.HTR_APC_EN_Bypass;

// NETWORK 5
GV_IL.HTR_CHAMBER_EN := GV_IL.SPLC_TO_PLC.HTR_CHAMBER_EN OR GV_IL.HTR_CHAMBER_EN_Bypass;

// NETWORK 6
GV_IL.HTR_FORLINE_EN := GV_IL.SPLC_TO_PLC.HTR_FORLINE_EN OR GV_IL.HTR_FORLINE_EN_Bypass;

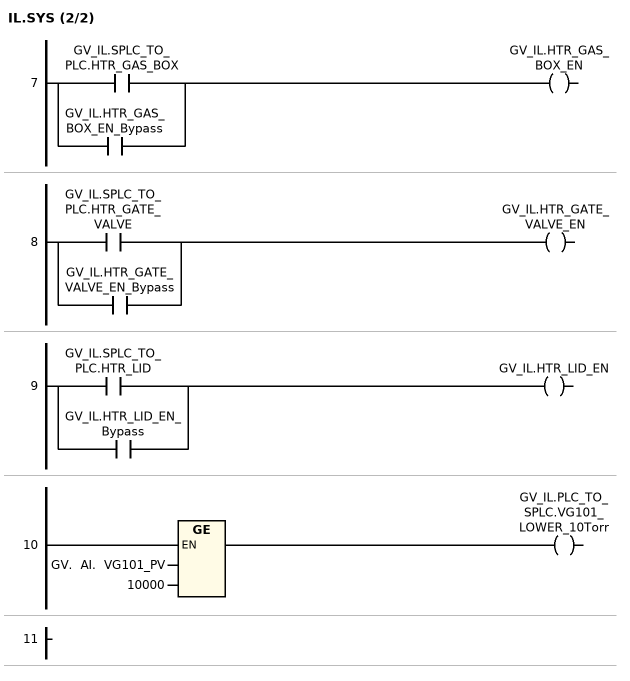
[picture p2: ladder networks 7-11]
// NETWORK 7
GV_IL.HTR_GAS_BOX_EN := GV_IL.SPLC_TO_PLC.HTR_GAS_BOX OR GV_IL.HTR_GAS_BOX_EN_Bypass;

// NETWORK 8
GV_IL.HTR_GATE_VALVE_EN := GV_IL.SPLC_TO_PLC.HTR_GATE_VALVE OR GV_IL.HTR_GATE_VALVE_EN_Bypass;

// NETWORK 9
GV_IL.HTR_LID_EN := GV_IL.SPLC_TO_PLC.HTR_LID OR GV_IL.HTR_LID_EN_Bypass;

// NETWORK 10
GV_IL.PLC_TO_SPLC.VG101_LOWER_10Torr := (GV.	AI.	VG101_PV) >= 10000;

// NETWORK 11
END_ACTION

ACTION Temp:
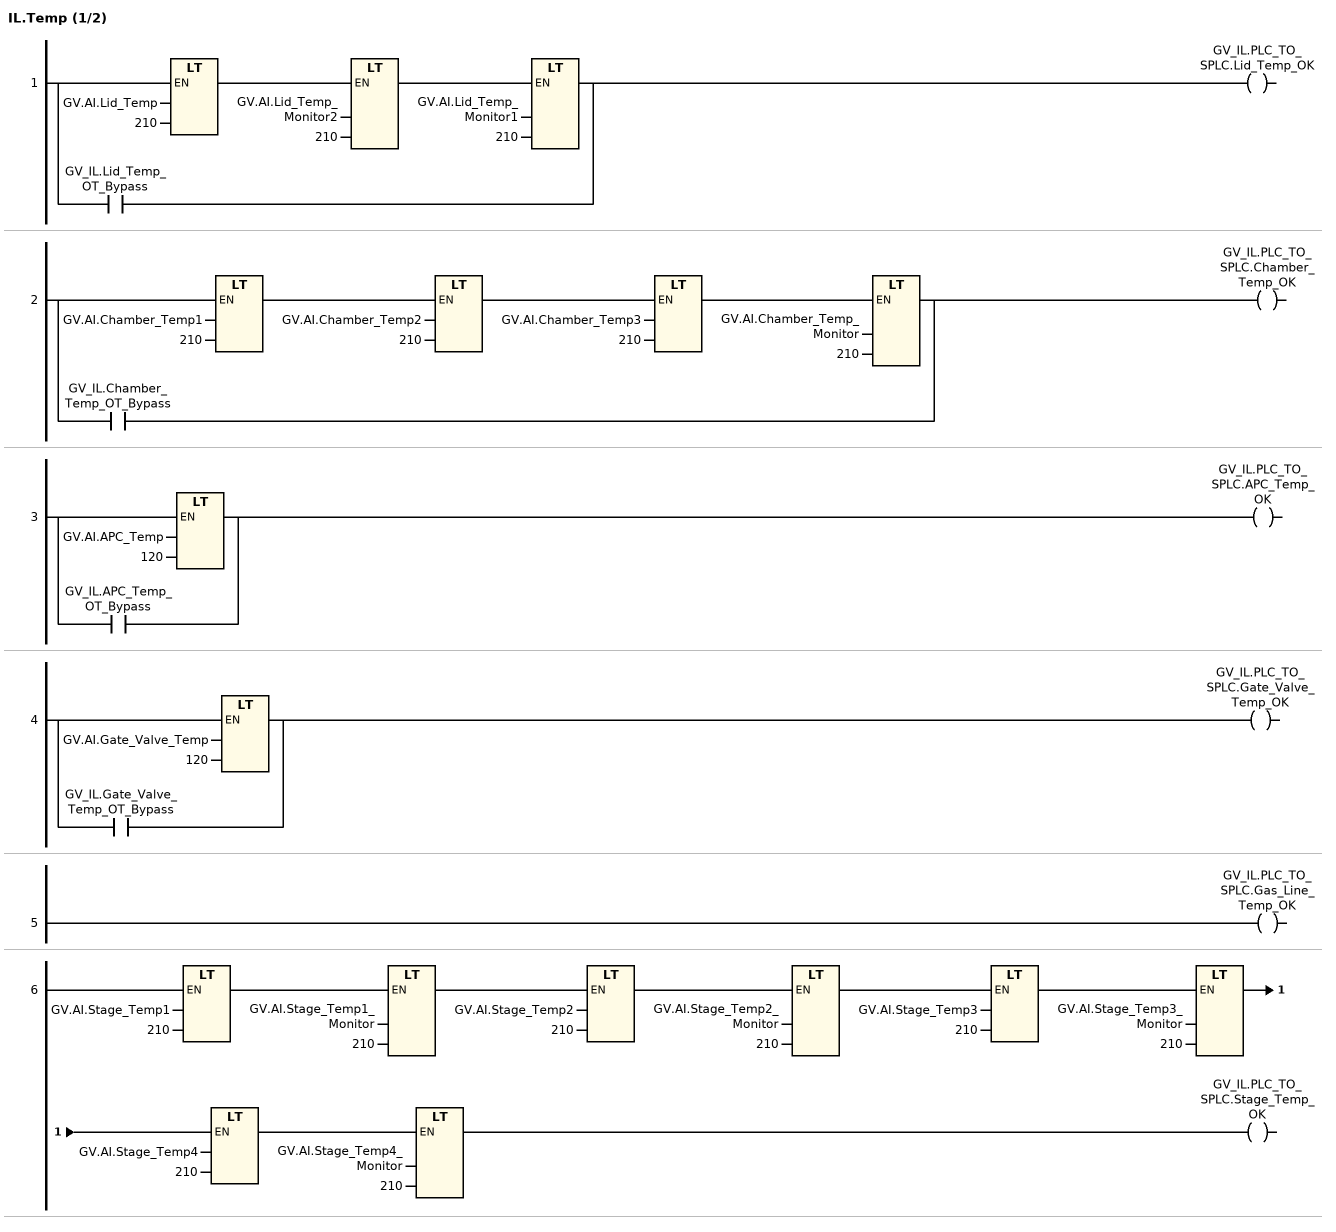
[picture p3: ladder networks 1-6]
// NETWORK 1
_w2 := GV_IL.Lid_Temp_OT_Bypass;
IF NOT _w2 THEN
    _w2 := GV.AI.Lid_Temp < 210 AND GV.AI.Lid_Temp_Monitor2 < 210 AND GV.AI.Lid_Temp_Monitor1 < 210;
END_IF
GV_IL.PLC_TO_SPLC.Lid_Temp_OK := _w2;

// NETWORK 2
_w3 := GV_IL.Chamber_Temp_OT_Bypass;
IF NOT _w3 THEN
    _w3 := GV.AI.Chamber_Temp1 < 210 AND GV.AI.Chamber_Temp2 < 210 AND GV.AI.Chamber_Temp3 < 210 AND GV.AI.Chamber_Temp_Monitor < 210;
END_IF
GV_IL.PLC_TO_SPLC.Chamber_Temp_OK := _w3;

// NETWORK 3
_w4 := GV_IL.APC_Temp_OT_Bypass;
IF NOT _w4 THEN
    _w4 := GV.AI.APC_Temp < 120;
END_IF
GV_IL.PLC_TO_SPLC.APC_Temp_OK := _w4;

// NETWORK 4
_w5 := GV_IL.Gate_Valve_Temp_OT_Bypass;
IF NOT _w5 THEN
    _w5 := GV.AI.Gate_Valve_Temp < 120;
END_IF
GV_IL.PLC_TO_SPLC.Gate_Valve_Temp_OK := _w5;

// NETWORK 5
GV_IL.PLC_TO_SPLC.Gas_Line_Temp_OK := TRUE;

// NETWORK 6
GV_IL.PLC_TO_SPLC.Stage_Temp_OK := GV.AI.Stage_Temp1 < 210 AND GV.AI.Stage_Temp1_Monitor < 210 AND GV.AI.Stage_Temp2 < 210 AND GV.AI.Stage_Temp2_Monitor < 210 AND GV.AI.Stage_Temp3 < 210 AND GV.AI.Stage_Temp3_Monitor < 210 AND GV.AI.Stage_Temp4 < 210 AND GV.AI.Stage_Temp4_Monitor < 210;

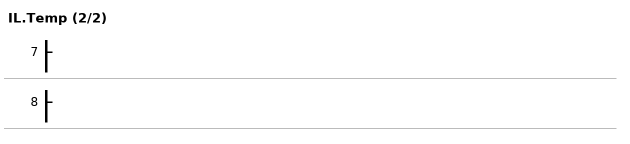
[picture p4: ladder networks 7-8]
// NETWORK 7

// NETWORK 8
END_ACTION

ACTION VALVE:
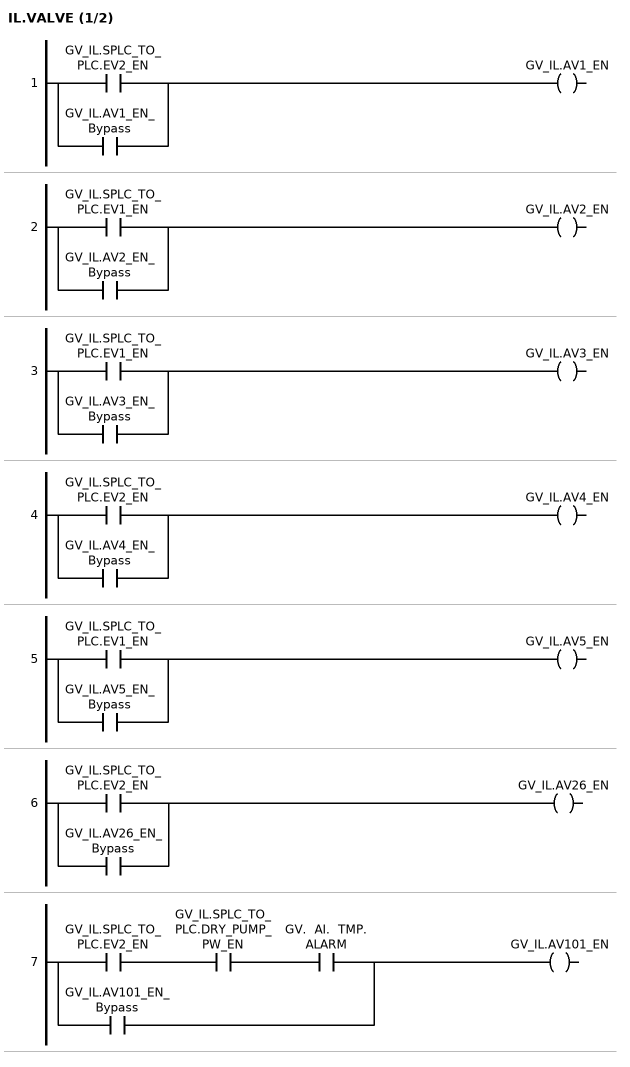
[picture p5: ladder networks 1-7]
// NETWORK 1
GV_IL.AV1_EN := GV_IL.SPLC_TO_PLC.EV2_EN OR GV_IL.AV1_EN_Bypass;

// NETWORK 2
GV_IL.AV2_EN := GV_IL.SPLC_TO_PLC.EV1_EN OR GV_IL.AV2_EN_Bypass;

// NETWORK 3
GV_IL.AV3_EN := GV_IL.SPLC_TO_PLC.EV1_EN OR GV_IL.AV3_EN_Bypass;

// NETWORK 4
GV_IL.AV4_EN := GV_IL.SPLC_TO_PLC.EV2_EN OR GV_IL.AV4_EN_Bypass;

// NETWORK 5
GV_IL.AV5_EN := GV_IL.SPLC_TO_PLC.EV1_EN OR GV_IL.AV5_EN_Bypass;

// NETWORK 6
GV_IL.AV26_EN := GV_IL.SPLC_TO_PLC.EV2_EN OR GV_IL.AV26_EN_Bypass;

// NETWORK 7
GV_IL.AV101_EN := GV_IL.SPLC_TO_PLC.EV2_EN AND GV_IL.SPLC_TO_PLC.DRY_PUMP_PW_EN AND (GV.	AI.	TMP.	ALARM) OR GV_IL.AV101_EN_Bypass;

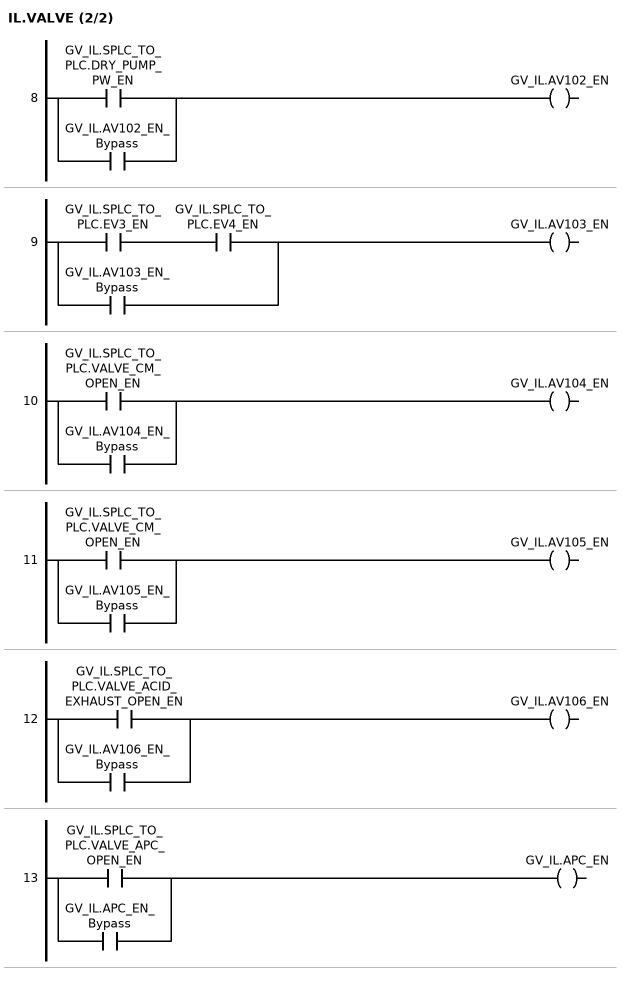
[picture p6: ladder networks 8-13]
// NETWORK 8
GV_IL.AV102_EN := GV_IL.SPLC_TO_PLC.DRY_PUMP_PW_EN OR GV_IL.AV102_EN_Bypass;

// NETWORK 9
GV_IL.AV103_EN := GV_IL.SPLC_TO_PLC.EV3_EN AND GV_IL.SPLC_TO_PLC.EV4_EN OR GV_IL.AV103_EN_Bypass;

// NETWORK 10
GV_IL.AV104_EN := GV_IL.SPLC_TO_PLC.VALVE_CM_OPEN_EN OR GV_IL.AV104_EN_Bypass;

// NETWORK 11
GV_IL.AV105_EN := GV_IL.SPLC_TO_PLC.VALVE_CM_OPEN_EN OR GV_IL.AV105_EN_Bypass;

// NETWORK 12
GV_IL.AV106_EN := GV_IL.SPLC_TO_PLC.VALVE_ACID_EXHAUST_OPEN_EN OR GV_IL.AV106_EN_Bypass;

// NETWORK 13
GV_IL.APC_EN := GV_IL.SPLC_TO_PLC.VALVE_APC_OPEN_EN OR GV_IL.APC_EN_Bypass;
END_ACTION

END_PROGRAM
